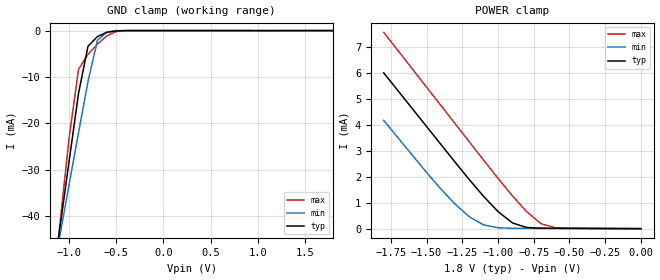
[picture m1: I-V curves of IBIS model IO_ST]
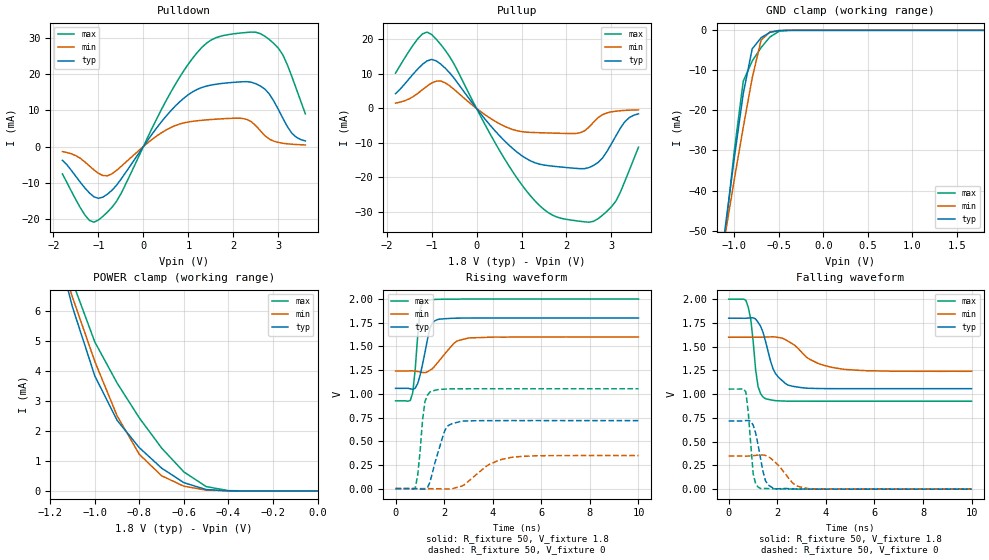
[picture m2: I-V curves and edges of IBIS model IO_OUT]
[IBIS Ver]   3.2
[Comment Char]   |_char
[File name]   sg5032can18.ibs
[File Rev]   1.0
[Date]   2015/11/24 22:00:00
[Source]
[Notes]
[Disclaimer]
This information is for modeling purposes only, and is not guaranteed.
Property of SEIKO EPSON Corp.,
unauthorized reproduction and/or distribution is strictly prohibited.
[Copyright]
Copyright 2006, SEIKO EPSON Corp.
[Component]   SG5032CAN
Si_location Pin
Timing_location Pin
[Manufacturer]   SEIKO EPSON Corp.
| COG
| COG
[Package]
R_pkg   56.75m   56.75m   56.75m
L_pkg   2.25n   2.25n   2.25n
C_pkg   0.860p   0.860p   0.860p
[Pin] signal_name   model_name
1   /ST   IO_ST
2   GND   GND
3   OUT   IO_OUT
4   Vcc   POWER
| Models and submodels in the file (2): IO_ST (Input), IO_OUT (3-state)
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[Model]   IO_ST
Model_type Input
Polarity Inverting
Vinh=1.44
Vinl=0.36
C_comp   5p   4p   6p
[Temperature Range] 25   105   -40
[Voltage Range]   1.8   1.6   2.0
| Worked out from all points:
|   GND clamp passes 1 mA (typ) near -0.67 V on its own axis
|   POWER clamp passes 1 mA (typ) near -1.06 V on its own axis
[GND Clamp]
-1.8V     -147.9mA   -125.7mA   -176.6mA
-1.2V     -57.55mA   -55.73mA   -61.1mA
-1.1V     -42.76mA   -44.37mA   -42.02mA
-1V       -28.06mA   -33.1mA    -23.01mA
-900mV    -13.48mA   -21.96mA   -8.306mA
-800mV    -3.366mA   -10.96mA   -5.116mA
-700mV    -1.291mA   -2.106mA   -2.915mA
-600mV    -372.2uA   -316.4uA   -1.132mA
-500mV    -49.71uA   -42.02uA   -183.2uA
-400mV    -3.647uA   -4.906uA   -9.881uA
1.8V      26.36pA    2.246uA    -5.957uA
[POWER Clamp]
-1.8V     6.002mA    4.172mA    7.564mA
-1.5V     3.935mA    2.165mA    5.451mA
-1.4V     3.247mA    1.528mA    4.746mA
-1.3V     2.558mA    941.9uA    4.042mA
-1.2V     1.881mA    452.2uA    3.338mA
-1.1V     1.238mA    141.7uA    2.633mA
-1V       658.8uA    35.17uA    1.938mA
-900mV    223.5uA    15.34uA    1.269mA
-800mV    44.81uA    11.29uA    656.6uA
-700mV    17.63uA    9.397uA    192.3uA
-600mV    13.19uA    7.818uA    34.43uA
0V        26.36pA    589.6pA    18.35pA
[Model]   IO_OUT
Model_type 3-state
Enable Active-High
Polarity Non-Inverting
Vmeas=0.90
C_comp   5p   4p   6p
[Temperature Range] 25   105   -40
[Voltage Range]   1.8   1.6   2.0
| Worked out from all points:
|   slope of the pulldown table from 0 to 0.27 V, typ, clamps not added: 57.2 ohm
|   slope of the pullup table from 0 to 0.27 V, typ, clamps not added: 61.8 ohm
|   GND clamp passes 1 mA (typ) near -0.64 V on its own axis
|   POWER clamp passes 1 mA (typ) near -0.74 V on its own axis
|   falling waveform, R_fixture 50, V_fixture 1.8: 20-80 % time 548ps typ, 1.16ns min, 265ps max; typ from 1.8 V to 1.06 V
|   falling waveform, R_fixture 50, V_fixture 0: 20-80 % time 334ps typ, 688ps min, 203ps max; typ from 0.718 V to 0 V
|   rising waveform, R_fixture 50, V_fixture 1.8: 20-80 % time 362ps typ, 715ps min, 213ps max; typ from 1.06 V to 1.8 V
|   rising waveform, R_fixture 50, V_fixture 0: 20-80 % time 484ps typ, 1.11ns min, 233ps max; typ from 0 V to 0.718 V
[Pullup]
-1.8V     4.269mA    1.545mA    10.26mA
-1.3V     11.53mA    4.429mA    20.29mA
-1V       14.21mA    7.346mA    21.46mA
-500mV    8.791mA    5.536mA    12.89mA
800mV     -11.57mA   -6.1mA     -18.27mA
1.3V      -15.77mA   -7.002mA   -26.84mA
1.8V      -16.9mA    -7.196mA   -31.57mA
2.3V      -17.48mA   -7.076mA   -32.74mA
2.8V      -14.41mA   -1.813mA   -30.98mA
3.1V      -7.93mA    -798.9uA   -26.84mA
3.3V      -3.806mA   -567.5uA   -21.05mA
3.6V      -1.553mA   -430.2uA   -11.23mA
[Pulldown]
-1.8V     -3.817mA   -1.401mA   -7.592mA
-1.2V     -12.86mA   -5.377mA   -20.44mA
-900mV    -14mA      -8.036mA   -19.32mA
-500mV    -9.088mA   -5.56mA    -13.08mA
300mV     5.224mA    2.946mA    7.777mA
900mV     13.39mA    6.542mA    21mA
1.3V      16.34mA    7.256mA    27.42mA
1.7V      17.38mA    7.633mA    30.46mA
2.4V      17.79mA    6.848mA    31.66mA
2.9V      12.54mA    1.469mA    28.5mA
3.3V      3.671mA    637.8uA    19.35mA
3.6V      1.529mA    439.7uA    9.045mA
[GND Clamp]
-1.8V     -177.4mA   -149.9mA   -210.3mA
-1.1V     -48.77mA   -50.63mA   -50.17mA
-1V       -31.82mA   -37.19mA   -29.98mA
-900mV    -15.78mA   -24.22mA   -12.71mA
-800mV    -4.669mA   -11.96mA   -7.684mA
-700mV    -1.852mA   -2.454mA   -4.316mA
-600mV    -505.1uA   -405.3uA   -1.654mA
-500mV    -63.64uA   -57.41uA   -272.4uA
-400mV    -4.376uA   -6.701uA   -15.57uA
1.8V      104.4pA    16.92nA    74.46pA
[POWER Clamp]
-1.8V     29.26mA    24.05mA    37.63mA
-1.2V     8.957mA    8.759mA    10.16mA
-1.1V     6.115mA    6.443mA    6.961mA
-1V       3.829mA    4.311mA    4.959mA
-900mV    2.354mA    2.501mA    3.593mA
-800mV    1.439mA    1.216mA    2.43mA
-700mV    759.3uA    504uA      1.427mA
-600mV    274.3uA    156.6uA    632.3uA
-500mV    45.05uA    27.63uA    144.7uA
-400mV    3.085uA    3.004uA    9.596uA
0V        104.3pA    706pA      107.3pA
[Falling Waveform]
R_fixture=50
V_fixture=1.8
V_fixture_min=1.6
V_fixture_max=2.0
0s        1.8V       1.6V       2V
707.1ps   1.8V       1.6V       1.989V
909.1ps   1.803V     1.6V       1.789V
1.212ns   1.755V     1.6V       1.077V
1.515ns   1.558V     1.601V     952.5mV
1.919ns   1.221V     1.603V     932.1mV
2.626ns   1.083V     1.53V      926.2mV
3.333ns   1.062V     1.368V     925.8mV
4.646ns   1.058V     1.265V     925.8mV
10ns      1.058V     1.241V     925.8mV
[Falling Waveform]
R_fixture=50
V_fixture=0
V_fixture_min=0
V_fixture_max=0
0s        717.6mV    348.9mV    1.054V
707.1ps   722.2mV    347.4mV    1.023V
808.1ps   722mV      348.3mV    806.4mV
1.01ns    672.2mV    352.7mV    160.2mV
1.313ns   322.1mV    359.7mV    6.462mV
1.515ns   88.29mV    354.9mV    6.876mV
1.919ns   2.251mV    281.9mV    2.729mV
2.727ns   1.675mV    46.09mV    488.1uV
3.333ns   462.7uV    3.266mV    129.9uV
10ns      -40.92uV   0V         6.061uV
[Rising Waveform]
R_fixture=50
V_fixture=1.8
V_fixture_min=1.6
V_fixture_max=2.0
0s        1.058V     1.241V     925.8mV
606.1ps   1.053V     1.242V     929.5mV
707.1ps   1.047V     1.242V     1.012V
1.01ns    1.195V     1.231V     1.889V
1.212ns   1.439V     1.224V     1.984V
1.515ns   1.748V     1.265V     1.994V
1.818ns   1.788V     1.356V     1.998V
2.424ns   1.798V     1.537V     2V
3.03ns    1.8V       1.59V      2V
10ns      1.8V       1.6V       2V
[Rising Waveform]
R_fixture=50
V_fixture=0
V_fixture_min=0
V_fixture_max=0
0s        0V         0V         0V
808.1ps   -942.5uV   205.4uV    5.883mV
909.1ps   -2.544mV   334.4uV    134.5mV
1.111ns   -5.397mV   319.8uV    725.1mV
1.212ns   -4.858mV   68.91uV    920.6mV
1.515ns   163.8mV    -1.212mV   1.03V
2.02ns    607.5mV    -3.406mV   1.05V
2.626ns   705.5mV    19.15mV    1.053V
4.747ns   717.7mV    328.6mV    1.054V
10ns      717.6mV    348.9mV    1.054V
[Ramp]
R_load=50
dV/dt_r   4.305E-1/4.780E-10   2.093E-1/1.109E-9   6.321E-1/2.269E-10
dV/dt_f   4.453E-1/5.452E-10   2.151E-1/1.152E-9   6.445E-1/2.601E-10
|[End   IO_OUT
